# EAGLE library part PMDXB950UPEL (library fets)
20 V 500mA, dual P-channel Trench MOSFET
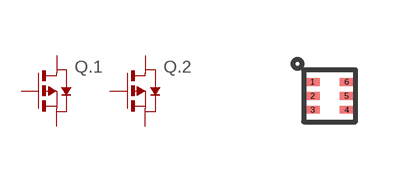
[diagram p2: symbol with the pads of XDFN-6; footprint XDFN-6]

Designator prefix Q; gates .1=P_MOSFET .2=P_MOSFET

## PMDXB950UPEL (DIGIKEY: 1727-2601-1-ND; MANUFACTURER: NEXPERIA; MPN: PMDXB950UPELZ)  [XDFN-6]
1  .1:S  pas
2  .1:G  pas
3  .2:D  pas
4  .2:S  pas
5  .2:G  pas
6  .1:D  pas

## Footprint XDFN-6 (pad centres in mm)
smd 0.35 x 0.2: 1 -0.425,0.35; 2 -0.425,0; 3 -0.425,-0.35; 4 0.425,-0.35; 5 0.425,0; 6 0.425,0.35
